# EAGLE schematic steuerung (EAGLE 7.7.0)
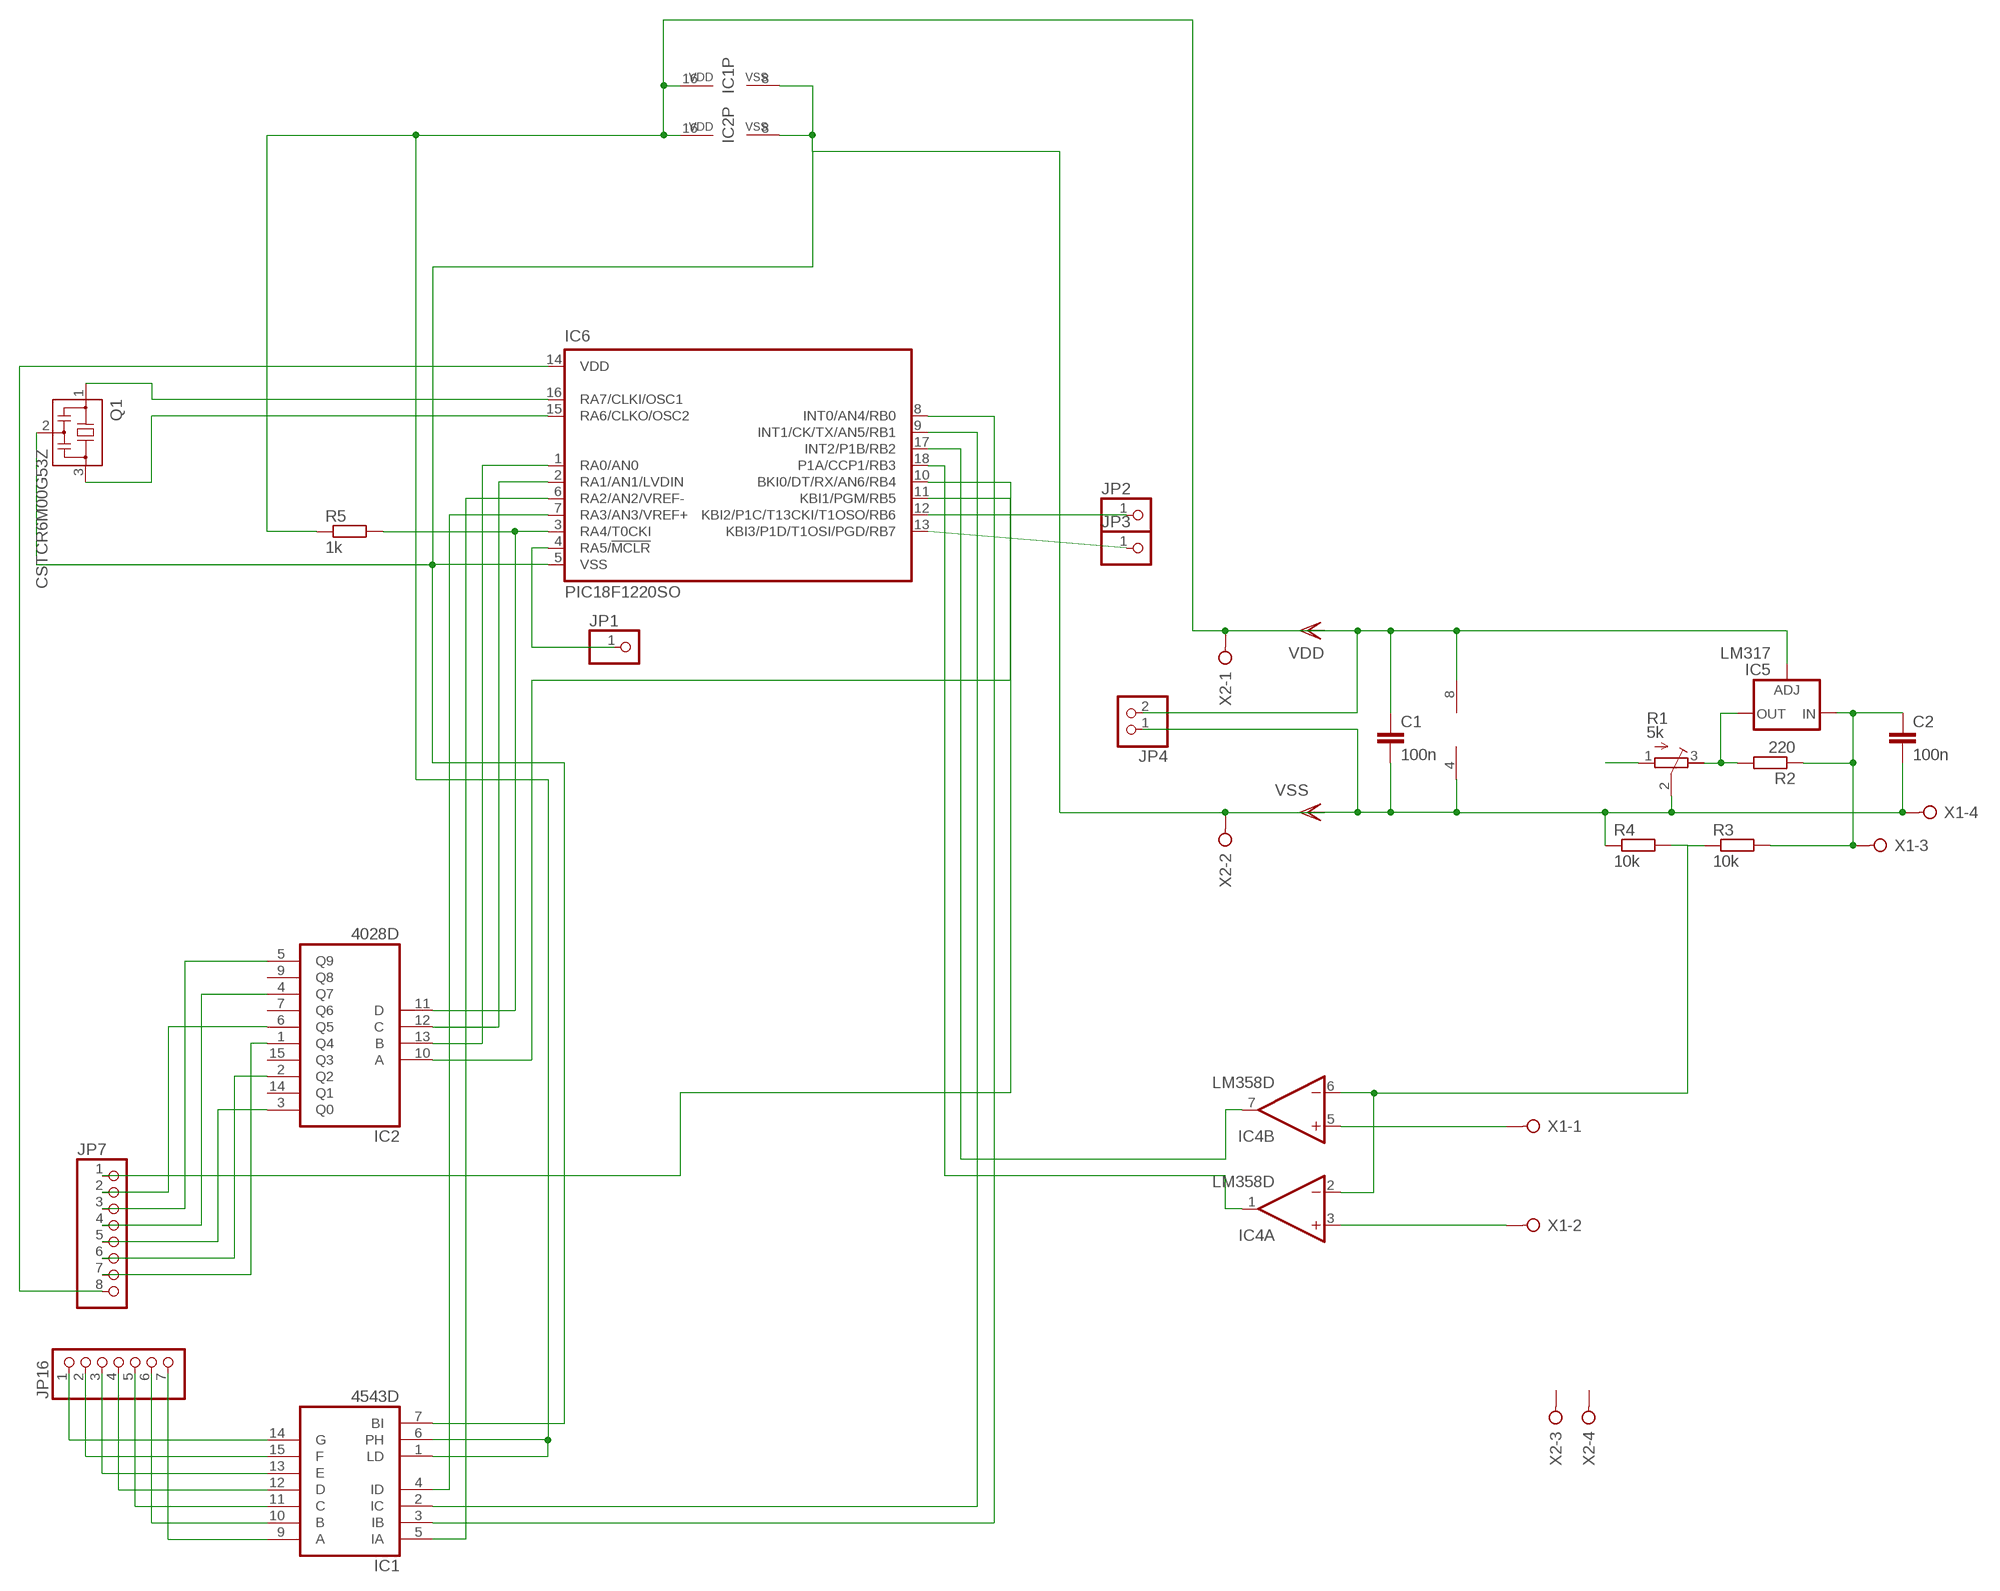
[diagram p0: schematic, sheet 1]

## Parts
C1  100n  C-EUC1206  [C1206]
C2  100n  C-EUC1206  [C1206]
IC1  4543D  [SO16]
IC2  4028D  [SO16]
IC4  LM358D  [SO08]
IC5  LM317  LM317MBSTT3  [SOT223]
IC6  PIC18F1220SO  [SO-18W]
JP1  PINHD-1X1  [1X01]
JP2  PINHD-1X1  [1X01]
JP3  PINHD-1X1  [1X01]
JP4  PINHD-1X2  [1X02]
JP7  PINHD-1X8  [1X08]
JP16  PINHD-1X7  [1X07]
Q1  CSTCR6M00G53Z  [CSTCR6M]
R1  5k  R-TRIMM3103  [RTRIM3103]
R2  220  R-EU_R1206  [R1206]
R3  10k  R-EU_R1206  [R1206]
R4  10k  R-EU_R1206  [R1206]
R5  1k  R-EU_R1206  [R1206]
X1  W237-04P  [W237-4P]
X2  W237-04P  [W237-4P]

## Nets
N$1: IC1.14(G) JP16.1
N$3: IC1.3(IB) IC6.8(INT0/AN4/RB0)
N$5: IC2.13(B) IC6.1(RA0/AN0)
N$6: IC6.14(VDD) JP7.8
N$7: IC2.5(Q9) JP7.3
N$9: C1.2 C2.2 IC1.7(BI) IC1.8(VSS) IC2.8(VSS) IC4.4(P:V-) IC6.5(VSS) JP4.1 Q1.2 R1.2(S) R4.1 X1.4 X2.2 ; supply symbol labelled VSS
N$11: IC4.2(A:-IN) IC4.6(B:-IN) R3.1 R4.2
N$14: IC2.3(Q0) JP7.5
N$16: IC2.1(Q4) JP7.7
N$17: IC2.6(Q5) JP7.2
N$20: IC1.9(A) JP16.7
N$21: IC1.15(F) JP16.2
N$23: IC1.10(B) JP16.6
N$24: IC1.11(C) JP16.5
N$25: IC4.5(B:+IN) X1.1
N$27: IC4.1(A:OUT) IC6.18(P1A/CCP1/RB3)
N$28: IC1.4(ID) IC6.7(RA3/AN3/VREF+)
N$29: IC1.12(D) JP16.4
N$32: IC1.2(IC) IC6.9(INT1/CK/TX/AN5/RB1)
N$34: IC6.15(RA6/CLKO/OSC2) Q1.3
N$35: IC5.4(OUT) R1.3(E) R2.2
N$36: R1.1(A)
N$40: IC1.13(E) JP16.3
N$49: IC2.2(Q2) JP7.6
N$60: IC2.11(D) IC6.3(RA4/T0CKI) R5.2
N$63: IC2.12(C) IC6.2(RA1/AN1/LVDIN)
N$70: IC4.7(B:OUT) IC6.17(INT2/P1B/RB2)
N$89: IC1.5(IA) IC6.6(RA2/AN2/VREF-)
N$96: C2.1 IC5.3(IN) R2.1 R3.2 X1.3
N$100: IC4.3(A:+IN) X1.2
N$101: IC2.4(Q7) JP7.4
N$111: IC2.10(A) IC6.11(KBI1/PGM/RB5)
N$120: IC6.4(RA5/!MCLR) JP1.1
N$124: IC6.10(BKI0/DT/RX/AN6/RB4) JP7.1
N$139: IC6.12(KBI2/P1C/T13CKI/T1OSO/RB6) JP2.1
N$163: IC6.13(KBI3/P1D/T1OSI/PGD/RB7) JP3.1
N$169: IC6.16(RA7/CLKI/OSC1) Q1.1
N$170: C1.1 IC1.1(LD) IC1.6(PH) IC1.16(VDD) IC2.16(VDD) IC4.8(P:V+) IC5.1(ADJ) JP4.2 R5.1 X2.1 ; supply symbol labelled VDD
Unconnected: IC2.7(Q6) IC2.9(Q8) IC2.14(Q1) IC2.15(Q3) X2.3 X2.4

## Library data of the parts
C1 C2 = resistor:C-EU: CAPACITOR, European symbol
IC1 = 45xx:4543: BCD to 7-segment LCD DECODER
IC2 = 40xx:4028: BCD to decimal DECODER
IC4 = linear:LM358: OP AMP also LM158; LM258; LM2904 Source: http://cache.national.com/ds/LM/LM158.pdf
IC5 = v-reg:LM317?*: 500 mA Adjustable Output Positive Voltage Regulator Source: http://www.onsemi.co.jp .. LM317M-D.PDF
IC6 = microchip:PIC18F1*20: 18/20/28-Pin High-Performance, Enhanced Flash Microcontrollers with 10-bit A/D and nanoWatt Technology Source: ww1.microchip.com/downloads/en/DeviceDoc/39605c.pdf; MF: MICROCHIP; MPN: PIC18F1220-I/SO; OC_FARNELL: 9761985; OC_NEWARK: 92C2430
JP1-JP3 = pinhead:PINHD-1X1: PIN HEADER
JP4 = pinhead:PINHD-1X2: PIN HEADER
JP7 = pinhead:PINHD-1X8: PIN HEADER
JP16 = pinhead:PINHD-1X7: PIN HEADER
Q1 = murata-filter:CSTCR: Resonator Source: murata.co.jp; MPN: CSTCR6M00G53-R0; OC_FARNELL: 1170434; OC_NEWARK: 25M8759
R1 = resistor:R-TRIMM: Trimm resistor
R2-R5 = resistor:R-EU_: RESISTOR, European symbol
X1 X2 = con-wago-508:W237-04P: WAGO SREW CLAMP; OC_FARNELL: unknown; OC_NEWARK: unknown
